FUNCTION CALL_READ_AI:VOID
TITLE = Ètení analogových vstupù

VAR_TEMP
  tRXIT : REAL ; //Odpadní hodnota
  tXIT  : BOOL ; //Odpadní BIT
END_VAR

BEGIN
NETWORK
TITLE = K04HJA10CR001XQ01
//Cteni AI:
//HOØÁK È.1 - VELIKOST PLAMENE 4-20mA
      CALL "READ_AIP" (
           PIW_IN                   := PIW   512,
           SRC                      := "DB_AIS".K04HJA10CR001XQ01,
           DST                      := "DB_AID".K04HJA10CR001XQ01);
      NOP 0;
NETWORK
TITLE = K04HJA20CR001XQ01
//Cteni AI:
//HOØÁK È.2 - VELIKOST PLAMENE 4-20mA
      CALL "READ_AIP" (
           PIW_IN                   := PIW   514,
           SRC                      := "DB_AIS".K04HJA20CR001XQ01,
           DST                      := "DB_AID".K04HJA20CR001XQ01);
      NOP 0;
NETWORK
TITLE = K04HJA30CR001XQ01
//Cteni AI:
//HOØÁK È.3 - VELIKOST PLAMENE 4-20mA
      CALL "READ_AIP" (
           PIW_IN                   := PIW   516,
           SRC                      := "DB_AIS".K04HJA30CR001XQ01,
           DST                      := "DB_AID".K04HJA30CR001XQ01);
      NOP 0;
NETWORK
TITLE = K04HJA40CR001XQ01
//Cteni AI:
//HOØÁK È.4 - VELIKOST PLAMENE 4-20mA
      CALL "READ_AIP" (
           PIW_IN                   := PIW   518,
           SRC                      := "DB_AIS".K04HJA40CR001XQ01,
           DST                      := "DB_AID".K04HJA40CR001XQ01);
      NOP 0;
NETWORK
TITLE = K04HHG36AS001XQ01
//Cteni AI:
//HOØÁK È.1 - POLOHA KLAPKY PLYNU
      CALL "READ_AIP" (
           PIW_IN                   := PIW   520,
           SRC                      := "DB_AIS".K04HHG36AS001XQ01,
           DST                      := "DB_AID".K04HHG36AS001XQ01);
      NOP 0;
NETWORK
TITLE = K04HHL11AS010XQ01
//Cteni AI:
//HOØÁK È.1 - POLOHA KLAPKY VZDUCHU
      CALL "READ_AIP" (
           PIW_IN                   := PIW   522,
           SRC                      := "DB_AIS".K04HHL11AS010XQ01,
           DST                      := "DB_AID".K04HHL11AS010XQ01);
      NOP 0;
NETWORK
TITLE = K04HHG37AS001XQ01
//Cteni AI:
//HOØÁK È.2 - POLOHA KLAPKY PLYNU
      CALL "READ_AIP" (
           PIW_IN                   := PIW   524,
           SRC                      := "DB_AIS".K04HHG37AS001XQ01,
           DST                      := "DB_AID".K04HHG37AS001XQ01);
      NOP 0;
NETWORK
TITLE = K04HHL71AS010XQ01
//Cteni AI:
//HOØÁK È.2 - POLOHA KLAPKY VZDUCHU
      CALL "READ_AIP" (
           PIW_IN                   := PIW   526,
           SRC                      := "DB_AIS".K04HHL71AS010XQ01,
           DST                      := "DB_AID".K04HHL71AS010XQ01);
      NOP 0;
NETWORK
TITLE = K04HHG38AS001XQ01
//Cteni AI:
//HOØÁK È.3 - POLOHA KLAPKY PLYNU
      CALL "READ_AIP" (
           PIW_IN                   := PIW   528,
           SRC                      := "DB_AIS".K04HHG38AS001XQ01,
           DST                      := "DB_AID".K04HHG38AS001XQ01);
      NOP 0;
NETWORK
TITLE = K04HHL51AS010XQ01
//Cteni AI:
//HOØÁK È.3 - POLOHA KLAPKY VZDUCHU
      CALL "READ_AIP" (
           PIW_IN                   := PIW   530,
           SRC                      := "DB_AIS".K04HHL51AS010XQ01,
           DST                      := "DB_AID".K04HHL51AS010XQ01);
      NOP 0;
NETWORK
TITLE = K04HHG39AS001XQ01
//Cteni AI:
//HOØÁK È.4 - POLOHA KLAPKY PLYNU
      CALL "READ_AIP" (
           PIW_IN                   := PIW   532,
           SRC                      := "DB_AIS".K04HHG39AS001XQ01,
           DST                      := "DB_AID".K04HHG39AS001XQ01);
      NOP 0;
NETWORK
TITLE = K04HHL31AS010XQ01
//Cteni AI:
//HOØÁK È.4 - POLOHA KLAPKY VZDUCHU
      CALL "READ_AIP" (
           PIW_IN                   := PIW   534,
           SRC                      := "DB_AIS".K04HHL31AS010XQ01,
           DST                      := "DB_AID".K04HHL31AS010XQ01);
      NOP 0;
NETWORK
TITLE = PIW536
//Cteni AI:
//REZERVA
      CALL "READ_AIP" (
           PIW_IN                   := PIW   536,
           SRC                      := "DB_AIS".PIW536,
           DST                      := "DB_AID".PIW536);
      NOP 0;
NETWORK
TITLE = PIW538
//Cteni AI:
//REZERVA
      CALL "READ_AIP" (
           PIW_IN                   := PIW   538,
           SRC                      := "DB_AIS".PIW538,
           DST                      := "DB_AID".PIW538);
      NOP 0;
NETWORK
TITLE = PIW540
//Cteni AI:
//REZERVA
      CALL "READ_AIP" (
           PIW_IN                   := PIW   540,
           SRC                      := "DB_AIS".PIW540,
           DST                      := "DB_AID".PIW540);
      NOP 0;
NETWORK
TITLE = PIW542
//Cteni AI:
//REZERVA
      CALL "READ_AIP" (
           PIW_IN                   := PIW   542,
           SRC                      := "DB_AIS".PIW542,
           DST                      := "DB_AID".PIW542);
      NOP 0;
END_FUNCTION
